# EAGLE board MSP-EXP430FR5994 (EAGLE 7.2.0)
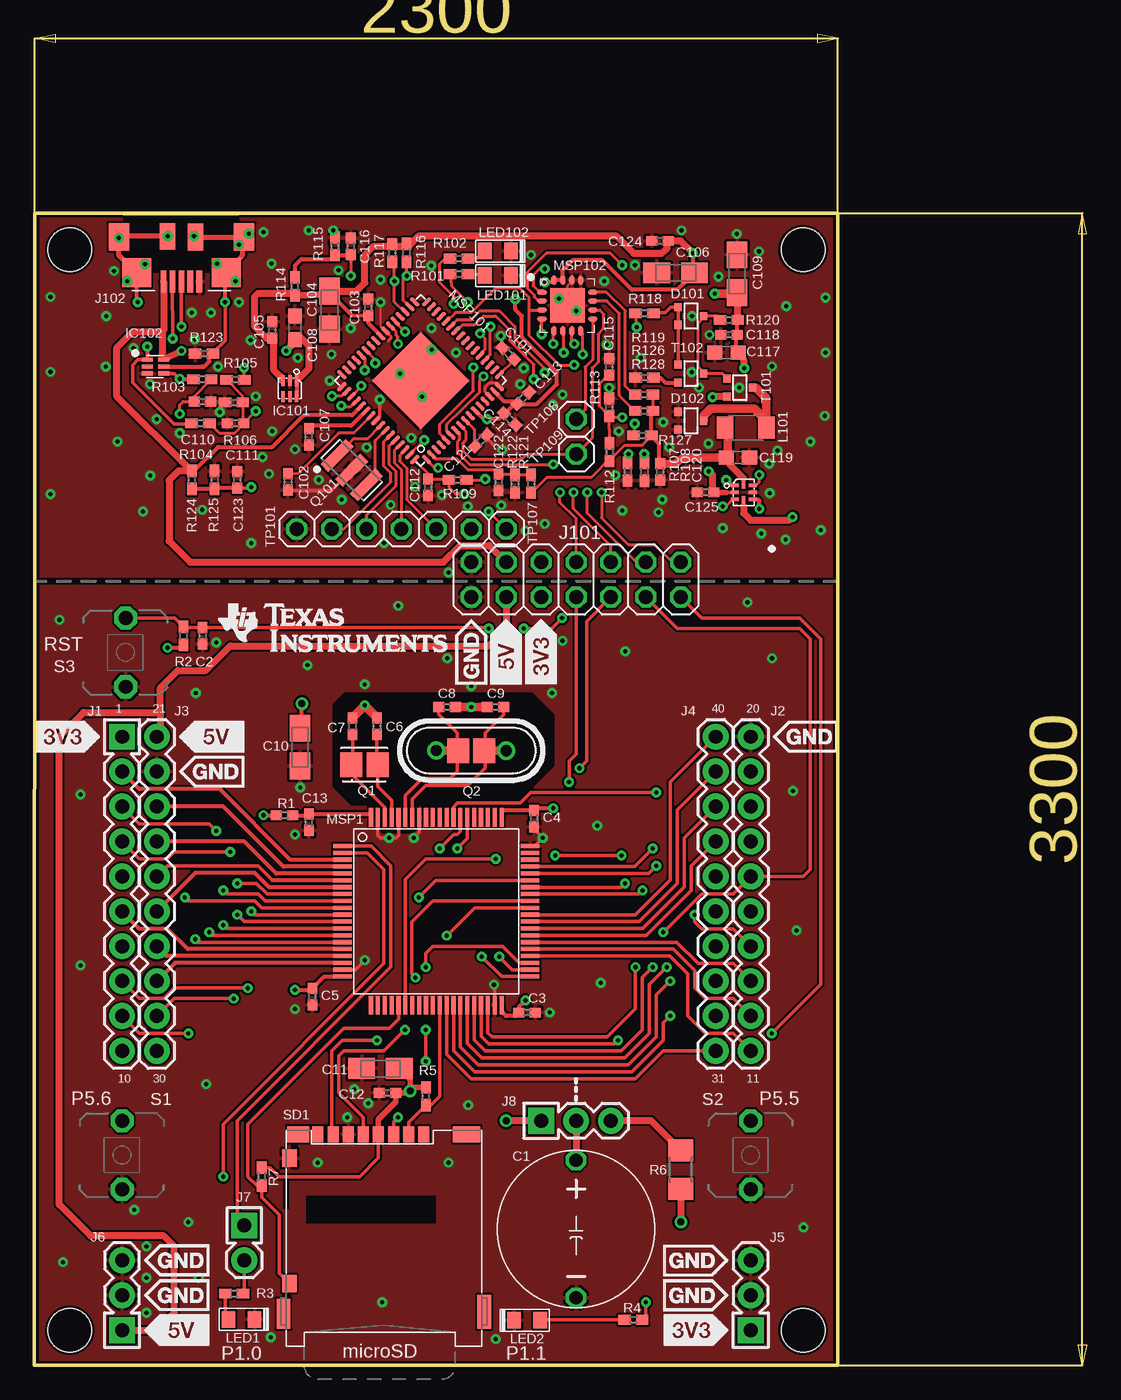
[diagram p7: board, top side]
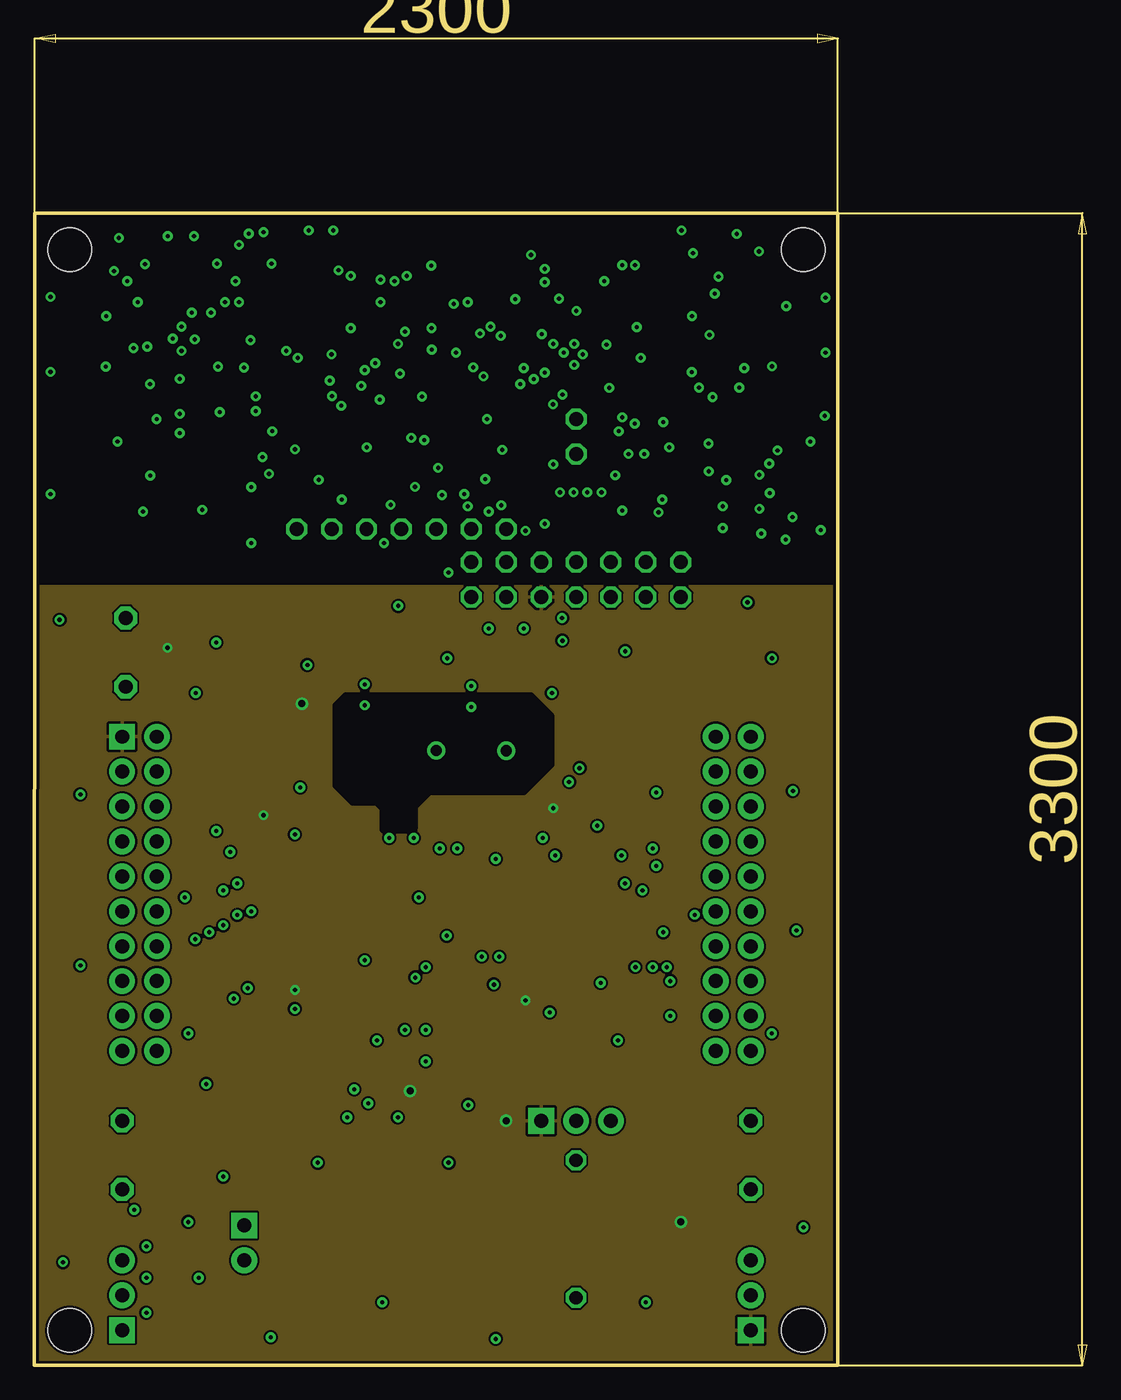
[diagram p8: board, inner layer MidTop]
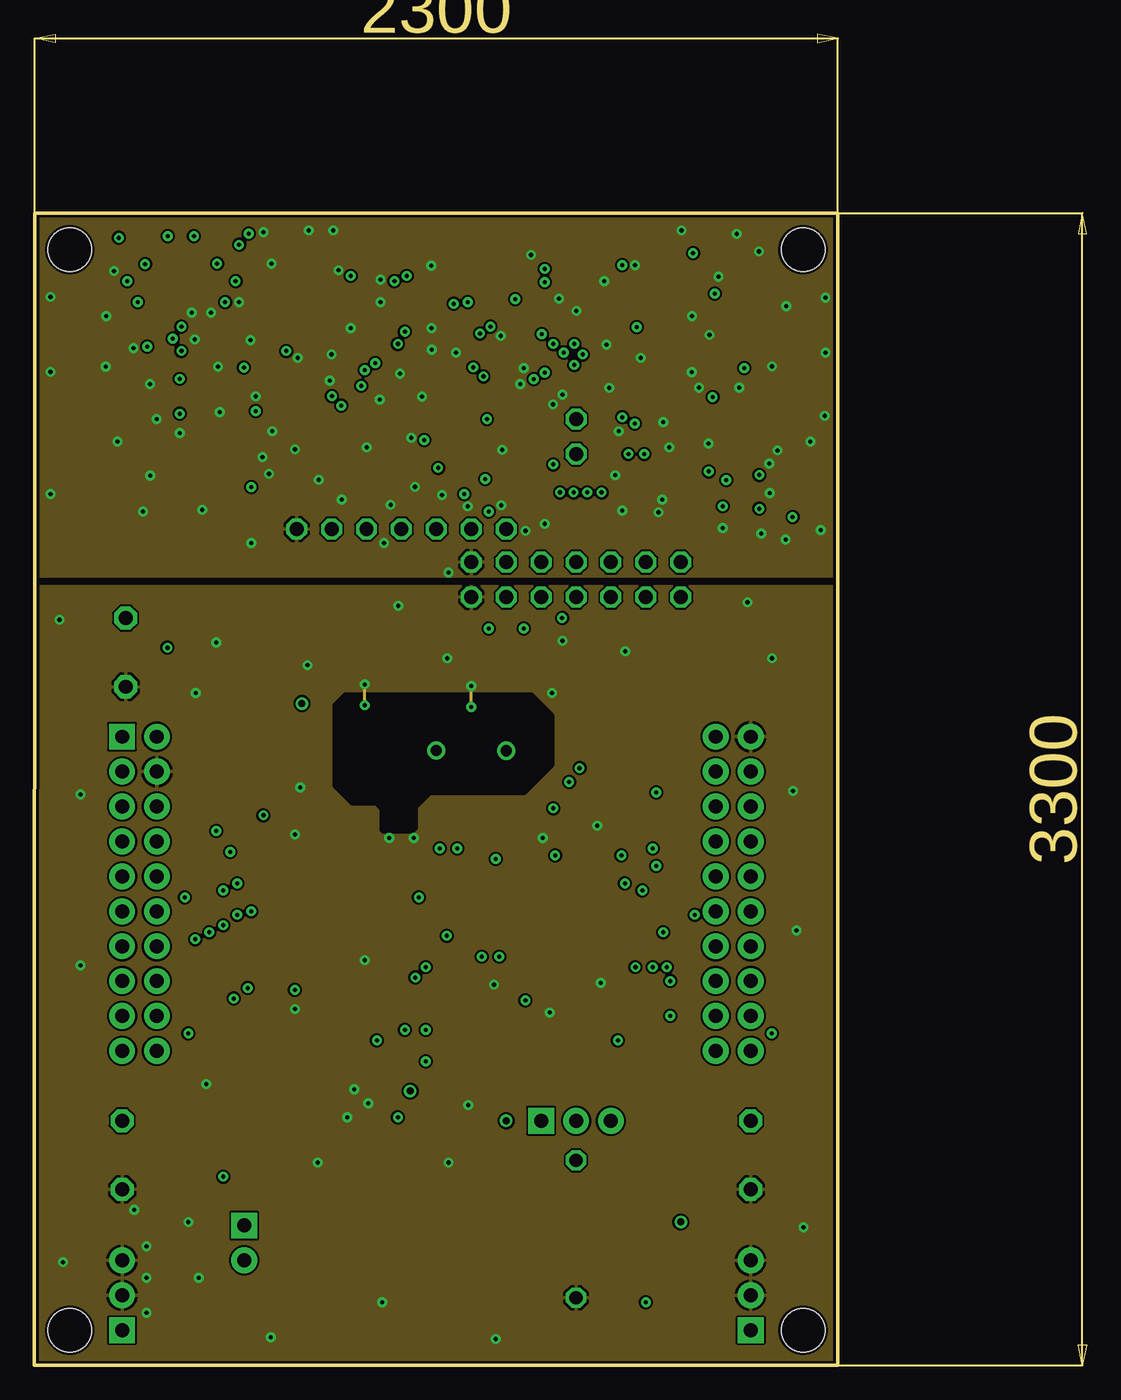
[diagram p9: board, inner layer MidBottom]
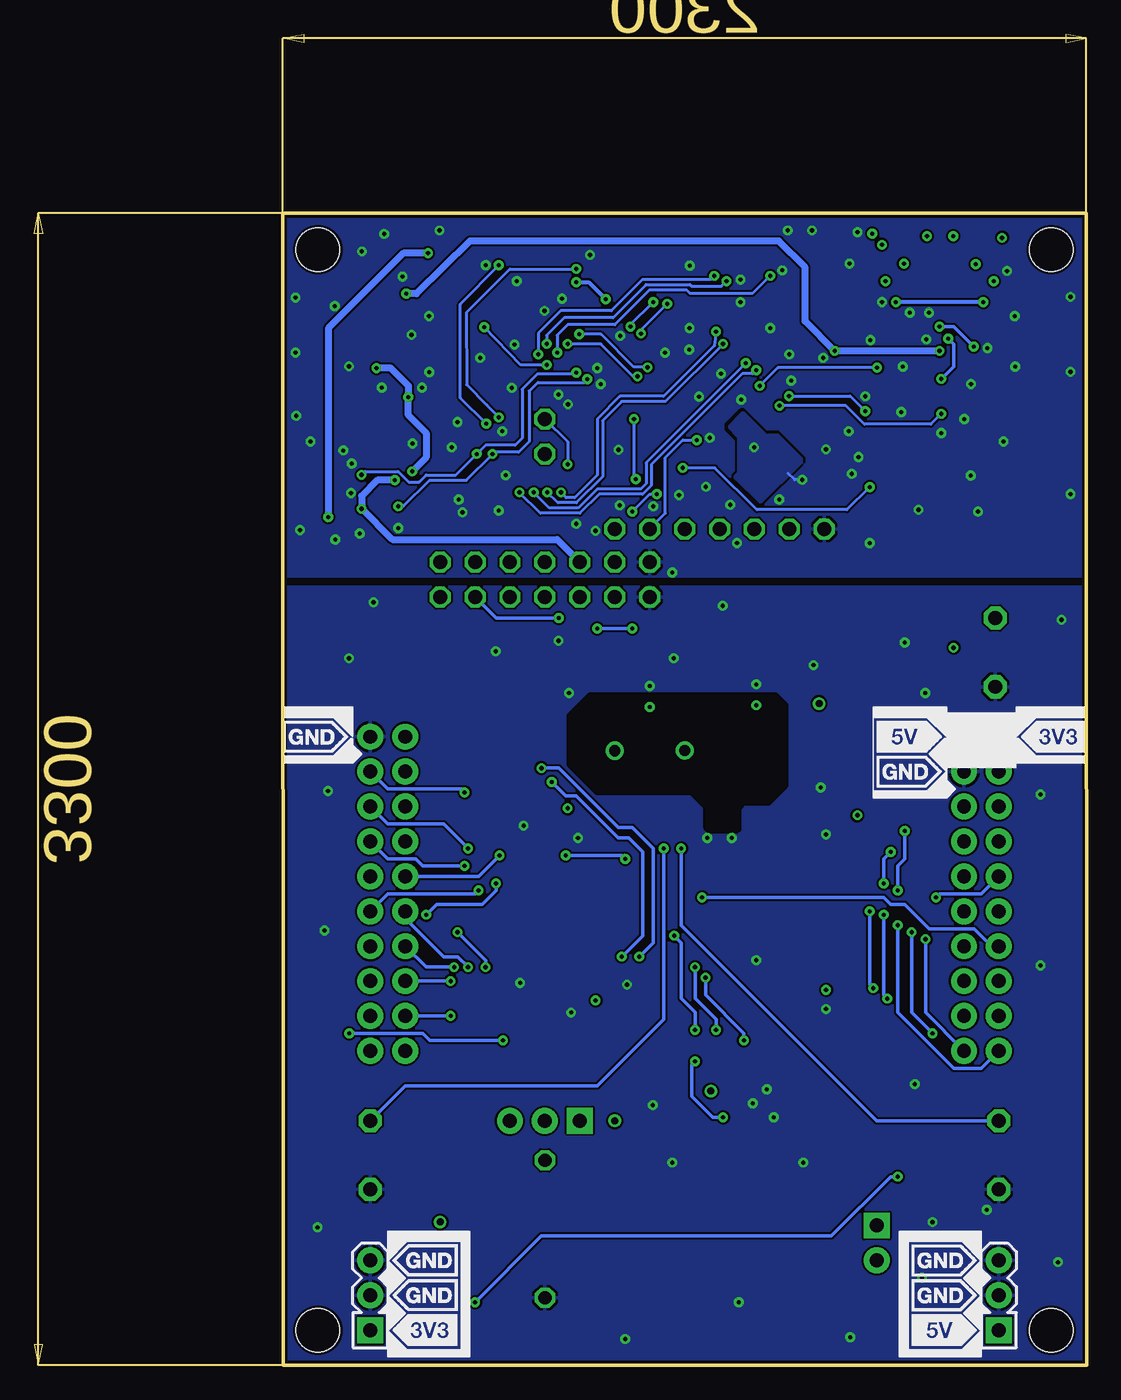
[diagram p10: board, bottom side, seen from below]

Size 76.53 x 96.82 mm. Coordinates in mm from the lower left corner, seen from the top.
Outline: 0,0 58.42,0 58.45,83.82 0.03,83.82 0,0
Copper layers (1+2*15+16): Top 0.0178mm / dielectric 12mil / MidTop 0.0356mm / dielectric 27mil / MidBottom 0.0356mm / dielectric 12mil / Bottom 0.0178mm
Design rules "MSP430 PCBExpress 4-layer-Stein": minimum track width 6mil, minimum drill 12mil, track to track 6mil, track to pad 6mil, pad to pad 6mil, via to via 8mil, smd to smd 6mil, copper to edge 8mil, drill to drill 8mil, minimum pad ring 10mil, minimum via ring 8mil, stop-mask expansion 8mil, vias tented up to drill 15mil, thermal gap 8mil
Net classes: 0 default: width 0.254 mm; 1 Ground: width 0.305 mm, drill 0.305 mm, clearance 0.152 mm to class 0, clearance 0.152 mm; 2 Power: width 0.406 mm, drill 0.305 mm, clearance 0.152 mm to class 0, clearance 0.152 mm to class 1, clearance 0.152 mm
tRestrict: area 20.5,62.5 to 26.3,69.6
bRestrict: area 20.5,62.5 to 26.3,69.6

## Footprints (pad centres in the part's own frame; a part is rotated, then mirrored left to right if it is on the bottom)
PANASONIC_SUPERCAP = drill 0.965 octagon: + 0,5; - 0,-5
0402 = smd 0.8 x 0.7: 1 -0.6,0; 2 0.6,0
A/3216-18R = smd 1.95 x 1.5: + 1.375,0; - -1.375,0
C0603 = smd 1.1 x 1: 1 -0.85,0; 2 0.85,0
SOT323 = smd 0.6 x 0.55: 1 -0.65,-0.825; 2 0.65,-0.825; 3 0,1.025
WSON_DSE = smd 0.25 x 0.8: 1 0,0; 2 0.5,0; 3 1,0; 5 0.5,1.15; 6 0,1.15; P4 1,1.15
SON(DRY)6 = smd 0.81 x 0.305: 1 -0.1,0; 2 -0.1,-0.5; 3 -0.1,-1; 4 1.1,-1; 5 1.1,-0.5; 6 1.1,0
UQFN_RSE = smd 0.25 x 0.58: 1 -0.5,-0.65; 2 0,-0.65; 3 0.5,-0.65; 5 0.5,0.65; 6 0,0.65; 7 -0.5,0.65 | smd 0.58 x 0.25: 4 0.55,0; 8 -0.55,0
J1 = drill 1.016 pad 1.88 square: 1 0,22.86 | drill 1.016 pad 1.88: 2 0,20.32; 3 0,17.78; 4 0,15.24; 5 0,12.7; 6 0,10.16; 7 0,7.62; 8 0,5.08; 9 0,2.54; 10 0,0
J2 = drill 1.016 pad 1.88: 11 0,0; 12 0,2.54; 13 0,5.08; 14 0,7.62; 15 0,10.16; 16 0,12.7; 17 0,15.24; 18 0,17.78; 19 0,20.32; 20 0,22.86
J3 = drill 1.016 pad 1.88: 21 0,22.86; 22 0,20.32; 23 0,17.78; 24 0,15.24; 25 0,12.7; 26 0,10.16; 27 0,7.62; 28 0,5.08; 29 0,2.54; 30 0,0
J4 = drill 1.016 pad 1.88: 31 0,0; 32 0,2.54; 33 0,5.08; 34 0,7.62; 35 0,10.16; 36 0,12.7; 37 0,15.24; 38 0,17.78; 39 0,20.32; 40 0,22.86
3PIN_PWR_3V3 = drill 1.016 pad 1.88 square: 1 0,0 | drill 1.016 pad 1.88: 2 0,2.54; 3 0,5.08
3PIN_PWR_5V = drill 1.016 pad 1.88 square: 1 0,0 | drill 1.016 pad 1.88: 2 0,2.54; 3 0,5.08
1X02 = drill 1.016 pad 1.88 square: 1 -1.27,0 | drill 1.016 pad 1.88: 2 1.27,0
1X03 = drill 1.016 pad 1.88 square: 1 0,0 | drill 1.016 pad 1.88: 2 2.54,0; 3 5.08,0
J101 = drill 1.016 octagon: 1 7.62,1.27; 2 7.62,-1.27; 3 5.08,1.27; 4 5.08,-1.27; 5 2.54,1.27; 6 2.54,-1.27; 7 0,1.27; 8 0,-1.27; 9 -2.54,1.27; 10 -2.54,-1.27; 11 -5.08,1.27; 12 -5.08,-1.27; 13 -7.62,1.27; 14 -7.62,-1.27
EZFET_UX62M-B-5P = smd 0.42 x 1.6: 1 1.3,1.3; 2 0.65,1.3; 3 0,1.3; 4 -0.65,1.3; 5 -1.3,1.3 | smd 2.1 x 2.1: S1 -3.25,0.65; S2 3.25,0.65 | smd 1.5 x 2: S3 -4.55,-1.95; S4 4.55,-1.95 | smd 1.144 x 1.949: S5 -1.016,-1.93; S6 1.016,-1.981
L3216C = smd 1.2 x 1.6: 1 -1.5,0; 2 1.5,0
LED0805 = smd 1 x 1.2: A 1.052,0.102; C -0.848,0.102
PN80 = smd 1.35 x 0.3: 1 -6.825,4.75; 2 -6.825,4.25; 3 -6.825,3.75; 4 -6.825,3.25; 5 -6.825,2.75; 6 -6.825,2.25; 7 -6.825,1.75; 8 -6.825,1.25; 9 -6.825,0.75; 10 -6.825,0.25; 11 -6.825,-0.25; 12 -6.825,-0.75; 13 -6.825,-1.25; 14 -6.825,-1.75; 15 -6.825,-2.25; 16 -6.825,-2.75; 17 -6.825,-3.25; 18 -6.825,-3.75; 19 -6.825,-4.25; 20 -6.825,-4.75; 41 6.825,-4.75; 42 6.825,-4.25; 43 6.825,-3.75; 44 6.825,-3.25; 45 6.825,-2.75; 46 6.825,-2.25; 47 6.825,-1.75; 48 6.825,-1.25; 49 6.825,-0.75; 50 6.825,-0.25; 51 6.825,0.25; 52 6.825,0.75; 53 6.825,1.25; 54 6.825,1.75; 55 6.825,2.25; 56 6.825,2.75; 57 6.825,3.25; 58 6.825,3.75; 59 6.825,4.25; 60 6.825,4.75 | smd 0.3 x 1.35: 21 -4.75,-6.825; 22 -4.25,-6.825; 23 -3.75,-6.825; 24 -3.25,-6.825; 25 -2.75,-6.825; 26 -2.25,-6.825; 27 -1.75,-6.825; 28 -1.25,-6.825; 29 -0.75,-6.825; 30 -0.25,-6.825; 31 0.25,-6.825; 32 0.75,-6.825; 33 1.25,-6.825; 34 1.75,-6.825; 35 2.25,-6.825; 36 2.75,-6.825; 37 3.25,-6.825; 38 3.75,-6.825; 39 4.25,-6.825; 40 4.75,-6.825; 61 4.75,6.825; 62 4.25,6.825; 63 3.75,6.825; 64 3.25,6.825; 65 2.75,6.825; 66 2.25,6.825; 67 1.75,6.825; 68 1.25,6.825; 69 0.75,6.825; 70 0.25,6.825; 71 -0.25,6.825; 72 -0.75,6.825; 73 -1.25,6.825; 74 -1.75,6.825; 75 -2.25,6.825; 76 -2.75,6.825; 77 -3.25,6.825; 78 -3.75,6.825; 79 -4.25,6.825; 80 -4.75,6.825
RGC64 = smd 0.825 x 0.28: 1 -4.36,3.75; 2 -4.36,3.25; 3 -4.36,2.75; 4 -4.36,2.25; 5 -4.36,1.75; 6 -4.36,1.25; 7 -4.36,0.75; 8 -4.36,0.25; 9 -4.36,-0.25; 10 -4.36,-0.75; 11 -4.36,-1.25; 12 -4.36,-1.75; 13 -4.36,-2.25; 14 -4.36,-2.75; 15 -4.36,-3.25; 16 -4.36,-3.75; 33 4.36,-3.75; 34 4.36,-3.25; 35 4.36,-2.75; 36 4.36,-2.25; 37 4.36,-1.75; 38 4.36,-1.25; 39 4.36,-0.75; 40 4.36,-0.25; 41 4.36,0.25; 42 4.36,0.75; 43 4.36,1.25; 44 4.36,1.75; 45 4.36,2.25; 46 4.36,2.75; 47 4.36,3.25; 48 4.36,3.75 | smd 0.28 x 0.825: 17 -3.75,-4.36; 18 -3.25,-4.36; 19 -2.75,-4.36; 20 -2.25,-4.36; 21 -1.75,-4.36; 22 -1.25,-4.36; 23 -0.75,-4.36; 24 -0.25,-4.36; 25 0.25,-4.36; 26 0.75,-4.36; 27 1.25,-4.36; 28 1.75,-4.36; 29 2.25,-4.36; 30 2.75,-4.36; 31 3.25,-4.36; 32 3.75,-4.36; 49 3.75,4.36; 50 3.25,4.36; 51 2.75,4.36; 52 2.25,4.36; 53 1.75,4.36; 54 1.25,4.36; 55 0.75,4.36; 56 0.25,4.36; 57 -0.25,4.36; 58 -0.75,4.36; 59 -1.25,4.36; 60 -1.75,4.36; 61 -2.25,4.36; 62 -2.75,4.36; 63 -3.25,4.36; 64 -3.75,4.36 | smd 5 x 5: TP 0,0
RSA16 = smd 0.7 x 0.35: 1 -1.85,0.975; 2 -1.85,0.325; 3 -1.85,-0.325; 4 -1.85,-0.975; 9 1.85,-0.975; 10 1.85,-0.325; 11 1.85,0.325; 12 1.85,0.975 | smd 0.35 x 0.7: 5 -0.975,-1.85; 6 -0.325,-1.85; 7 0.325,-1.85; 8 0.975,-1.85; 13 0.975,1.85; 14 0.325,1.85; 15 -0.325,1.85; 16 -0.975,1.85 | smd 2.5 x 2.5: TP 0,0
LF_CRYSTAL = smd 1.778 x 1.6: 1 0,0.94; 2 0,-0.965
HF_XTAL = drill 0.813: 1 0.009,2.543; 2 -0.001,-2.533 | smd 1.8 x 1.6: P$1 0,-0.95; P$2 0,0.95
CSTCR4M = smd 0.8 x 2.6: 1 -1.5,0; 2 0,0; 3 1.5,0
0402' = smd 0.9 x 0.7: 1 -0.65,0; 2 0.65,0
R3216 = smd 1.6 x 1.8: 1 -1.4,0; 2 1.4,0
PBTH = drill 1.016 pad 1.676 octagon: 1 -0.001,0.001; 2 5.001,0.001
SD-502702-003 = smd 0.8 x 1.16: 1 -2.9,-17.82; 2 -1.8,-17.82; 3 -0.7,-17.82; 4 0.4,-17.82; 5 1.5,-17.82; 6 2.6,-17.82; 7 3.7,-17.82; 8 4.8,-17.82 | smd 1.05 x 1.25: A 6.885,-16.075; B 6.885,-6.95 | smd 1 x 2.5: P$9 -7.3,-4.9 | smd 1 x 2.2: P$10 7.3,-4.75 | smd 2 x 1.16: P$11 -6.01,-17.82 | smd 1.6 x 1.16: P$12 6.24,-17.82
1X01 = drill 1.016 octagon: 1 0,0
MOUNTHOLE_125MIL = hole 3.175: 0,0

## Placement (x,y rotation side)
C1  0.1F  [PANASONIC_SUPERCAP]  39.4,9.91 0 top
C2  1n  [0402]  12.24,53.07 270 top
C3  100n  [0402]  35.84,25.65 0 top
C4  100n  [0402]  36.35,39.75 270 top
C5  100n  [0402]  20.22,26.8 270 top
C6  22p  [0402]  24.92,46.48 90 top
C7  22p  [0402]  23.14,46.48 90 top
C8  DNP  [0402]  30,47.88 0 top
C9  DNP  [0402]  33.55,47.88 180 top
C10  10u  [A/3216-18R]  19.33,44.96 90 top
C11  1u  [A/3216-18R]  25.17,21.59 0 top
C12  100n  [0402]  25.68,19.81 180 top
C13  100n  [0402]  19.96,39.5 270 top
C101  470n  [0402]  34.46,73.6 135 top
C102  220n  [0402]  18.44,64.26 270 top
C103  100n  [0402]  24.28,76.96 90 top
C104  10u  [A/3216-18R]  21.46,76.76 90 top
C105  100n  [0402]  17.3,75.31 90 top
C106  4.7u  [A/3216-18R]  46.63,79.47 0 top
C107  220n  [0402]  19.96,67.54 270 top
C108  1u  [C0603]  18.95,75.46 90 top
C109  4.7u  [A/3216-18R]  51.11,79.4 270 top
C110  10p  [0402]  12.22,70.1 0 top
C111  10p  [0402]  14.63,68.52 180 top
C112  1n  [0402]  28.64,63.85 270 top
C113  100n  [0402]  35.55,70.36 45 top
C114  100n  [0402]  34.57,68.83 315 top
C115  33p  [0402]  41.81,72.64 270 top
C116  33p  [0402]  23.01,81.41 270 top
C117  4.7u  [C0603]  50.33,73.67 180 top
C118  100n  [0402]  50.51,74.97 180 top
C119  4.7u  [C0603]  51.16,66.03 0 top
C120  100n  [0402]  45.52,64.99 270 top
C121  100n  [0402]  32.48,67.26 45 top
C122  33p  [0402]  33.77,64.21 90 top
C123  33p  [0402]  14.76,64.41 270 top
C124  100n  [0402]  45.49,81.79 180 top
C125  100n  [0402]  48.79,63.5 180 top
D101  BAS40-05  [SOT323]  47.65,76.33 270 top
D102  BAS40-05  [SOT323]  47.65,68.71 270 top
DRAW1  [LOGO-ROCKET-10X7MM-BRD]  2.84,63.13 56 top
DRAW3  [LOGO-ROCKET-10X7MM-BRD]  10.52,15.59 7 top
IC101  [WSON_DSE]  19.08,71.63 180 top
IC102  TPD4E004DRYR  [SON(DRY)6]  8.31,73.15 0 top
IC103  TS5A21366RSER  [UQFN_RSE]  51.59,63.5 270 top
J1  BP_HEADERS_J1  [J1]  6.38,22.86 0 top
J2  BP_HEADERS_J2  [J2]  52.1,22.86 0 top
J3  BP_HEADERS_J3  [J3]  8.92,22.86 0 top
J4  BP_HEADERS_J4  [J4]  49.56,22.86 0 top
J5  HEADER 1X03  [3PIN_PWR_3V3]  52.1,2.54 0 bottom
J6  BP_HEADERS_PWR_5V  [3PIN_PWR_5V]  6.38,2.54 0 bottom
J7  JUMPER1X02  [1X02]  15.27,8.89 270 top
J8  JUMPER1X03  [1X03]  36.86,17.78 0 top
J101  J101_2X7_HEADER  [J101]  39.4,57.15 0 top
J102  Micro-USB  [EZFET_UX62M-B-5P]  10.69,80.14 180 top
L101  2u2  [L3216C]  51.73,68.19 180 top
LED1  Red  [LED0805]  15.16,3.43 180 top
LED2  Green  [LED0805]  35.74,3.17 0 top
LED101  Red  [LED0805]  33.81,79.38 180 top
LED102  Green  [LED0805]  33.81,81.15 180 top
MSP1  MSP430FR5994  [PN80]  29.24,33.02 0 top
MSP101  MSP430F5528IRGC  [RGC64]  28.09,71.63 135 top
MSP102  MSP430G2452IRSA16R  [RSA16]  38.76,77.09 0 top
Q1  LF_CRYSTAL  [LF_CRYSTAL]  24.03,43.69 270 top
Q2  [HF_XTAL]  31.78,44.7 90 top
Q101  PIEZO_CSTCR4M00G15L99  [CSTCR4M]  23.08,65.11 315 top
R1  0R  [0402]  18.19,40.01 0 top
R2  47k  [0402']  10.84,53.07 270 top
R3  470  [0402']  14.53,5.21 180 top
R4  390  [0402']  43.56,3.3 180 top
R5  47k  [0402']  28.47,19.56 90 top
R6  22  [R3216]  47.02,14.22 90 top
R7  DNP- 100k  [0402']  16.54,13.72 270 top
R101  470  [0402']  30.89,79.38 180 top
R102  390  [0402']  30.89,80.5 180 top
R103  27  [0402']  12.22,71.72 0 top
R104  27  [0402']  12.09,68.52 0 top
R105  1k4  [0402']  14.63,71.69 0 top
R106  1M  [0402']  14.5,70.04 180 top
R107  47k  [0402']  43.15,65 270 top
R108  47k  [0402']  44.37,65 270 top
R109  47k  [0402']  30.79,64.4 0 top
R112  220k  [0402']  41.84,66.42 90 top
R113  220k  [0402']  41.81,69.7 90 top
R114  220k  [0402']  18.95,78.49 90 top
R115  220k  [0402']  21.87,81.41 90 top
R116  4k7  [0402']  27.06,80.91 270 top
R117  4k7  [0402']  26.03,80.91 270 top
R118  820  [0402']  44.37,76.52 180 top
R119  0  [0402']  44.37,71.84 180 top
R120  470  [0402']  50.51,76.03 180 top
R121  220k  [0402']  36.13,64.14 90 top
R122  220k  [0402']  34.95,64.14 270 top
R123  33k  [0402']  12.34,73.6 180 top
R124  240k  [0402']  11.46,64.41 270 top
R125  150k  [0402']  13.11,64.41 90 top
R126  2k2  [0402']  44.35,70.61 180 top
R127  3k3  [0402']  44.22,67.64 180 top
R128  6k8  [0402']  44.35,69.42 180 top
S1  [PBTH]  6.38,17.78 270 top
S2  [PBTH]  52.1,17.78 270 top
S3  [PBTH]  6.63,54.36 270 top
SD1  SD-502702-003-1  [SD-502702-003]  25.43,-1.02 180 top
T101  DMG1013UW  [SOT323]  51.21,71.12 270 top
T102  BC850CW-115  [SOT323]  47.65,72.14 270 top
TP101  TEST_PIN2  [1X01]  19.08,60.83 0 top
TP102  TEST_PIN2  [1X01]  21.62,60.83 0 top
TP103  TEST_PIN2  [1X01]  24.16,60.83 0 top
TP104  TEST_PIN2  [1X01]  26.7,60.83 0 top
TP105  TEST_PIN2  [1X01]  29.24,60.83 0 top
TP106  TEST_PIN2  [1X01]  31.78,60.83 0 top
TP107  TEST_PIN2  [1X01]  34.32,60.83 0 top
TP108  TEST_PIN2  [1X01]  39.4,68.83 0 top
TP109  TEST_PIN2  [1X01]  39.4,66.29 0 top
U$1  FR5994_REARSILK_REV1_0  [FR5994_REARSILK_REV1_0]  0.03,0 0 top
U$2  MOUNTHOLE_125MIL  [MOUNTHOLE_125MIL]  2.57,2.54 0 top
U$3  MOUNTHOLE_125MIL  [MOUNTHOLE_125MIL]  2.57,81.15 0 top
U$4  [LOGO16_TPLACE]  13.28,51.73 0 top
U$5  MOUNTHOLE_125MIL  [MOUNTHOLE_125MIL]  55.91,2.54 0 top
U$6  MOUNTHOLE_125MIL  [MOUNTHOLE_125MIL]  55.91,81.15 0 top
U$7  MIKE_TM  [MIKE_TM]  25.17,8.13 0 top
U$8  BP_3PIN_SILK  [3PIN_PWR_SILK]  7.65,0.61 0 top
U$10  BP_3PIN_SILK_RT  [3PIN_PWR_SILK_RT]  50.83,0.61 0 top

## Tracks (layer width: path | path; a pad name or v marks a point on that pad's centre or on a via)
!RST!/SBWTDIO  (via drill 0.3)
  Top 0.203: R2.1 10.9,53.67
  Top 0.254: R2.1 10.2,54.36 S3.1 | 10.9,53.67 C2.1 32.97,53.67 v33.05,53.59 | v35.59,53.59 37.62,53.59 v38.38,54.36 | J101.4 46.76,53.59 55.65,53.59 56.41,52.83 56.41,36.07 55.91,35.56 J2.16 50.83,34.29 48.54,34.29 v45.75,31.5 | MSP1.38 32.99,24.19 33.3,23.88 41.68,23.88 43.71,25.91 v43.71,28.96
  Bottom 0.254: v33.05,53.59 v35.59,53.59 | v38.38,54.36 42.95,54.36 J101.4 | v43.71,28.96 43.71,29.46 v45.75,31.5
+3V3  (via drill 0.3, 0.51)
  Top 0.203: 10.84,52.35 R2.2
  Top 0.254: SD1.4 25.03,15.09 23.65,13.72 17.81,13.72 17.16,14.37 R7.1
  Top 0.305: v9.68,52.2 10.62,52.2 R2.2 | 33.99,25.91 MSP1.40 33.99,25.73 34.32,25.4 34.99,25.4 C3.1 35.24,26.07 v35.71,26.54 | v18.95,27.3 20.22,27.3 C5.1 21.09,28.27 MSP1.20 | MSP1.61 33.99,40.35 C4.1 36.35,40.51 v37.74,40.51 | v16.66,40.01 R1.1 | C10.+ 19.46,46.33 v19.46,48.13
  Top 0.406: J1.1 6.38,45.64 | R5.2 27.6,20.21 v27.33,19.94 | SD1.4 25.03,17.89 26.28,19.14 C12.1 27.2,19.81 v27.33,19.94 | 27.33,20.28 v27.33,19.94 | C11.+ 27.33,20.81 v27.33,19.94
  Top 0.508: R6.1 v47.02,10.41 | J8.1 v34.32,17.78
  pour MidTop: 0.03,56.64 0.03,0 58.45,0 58.45,56.64
+5V
  Top 0.508: J101.12 34.32,53.59 33.05,52.32 14.25,52.32 12.47,50.55 10.44,50.55 9.17,49.28 9.17,47.5 | J6.1 8.92,2.54 10.19,3.81 10.19,8.64 9.42,9.4 4.09,9.4 1.8,11.68 1.8,45.72 3.58,47.5 9.17,47.5 | 9.17,47.5 9.17,45.97 J3.21
EZFET_AVBUS  (via drill 0.3)
  Top 0.203: v29.36,65.28 29.11,65.28 28.52,65.86 MSP101.1
  Top 0.254: C123.2 15.71,63.81 v15.77,63.88
  Top 0.305: 12.96,63.86 12.98,63.88 13.12,63.88 | 13.11,63.86 R125.1 | 13.23,63.88 13.12,63.88 | 13.12,63.88 R125.1 | R124.2 R125.1 | R125.1 | C123.2 13.16,63.81 R125.1
  Bottom 0.203: v29.36,65.28 27.03,65.28 23.98,62.23 17.42,62.23 v15.77,63.88
EZFET_AVCC  (via drill 0.3)
  Top 0.152: 38.51,75.17 38.51,75.18 MSP102.6
  Top 0.203: 23.01,80.38 v23.01,79.25 | v38.51,73.66 38.51,75.17
  Top 0.305: 23.01,80.38 C116.2 | 22.97,80.48 23.01,80.52 23.01,80.48 | 23.01,80.39 23.01,80.48 | 23.01,80.48 C116.2 | R114.2 18.95,79.04 18.95,80.01 19.41,80.48 21.59,80.48 R115.1 22.96,80.76 C116.2
  Bottom 0.203: v23.01,79.25 24.28,77.98 28.85,77.98 29.11,78.23 31.78,78.23 34.32,75.69 37.74,75.69 38.51,74.93 v38.51,73.66
EZFET_AVCCOUT  (via drill 0.3)
  Top 0.152: 36.73,78.11 36.86,78.11 MSP102.1
  Top 0.203: R113.1 41.81,68.08 41.81,68.07 41.81,67.06 41.83,67.06 R112.2 | R113.1 42.03,68.96 v42.75,68.96 | 36.73,78.11 36.27,78.54 36.27,79.3 36.73,79.76 v37.11,79.76 | 41.78,72.06 41.78,72.03 41.83,71.98 41.83,71.99 41.86,72.01 | 41.86,71.92 41.86,72.01 | 41.86,72.01 41.86,72.04 41.83,72.06 | C115.2 41.79,72.09 41.07,71.37 41.07,69.8 41.68,69.19 41.77,68.94 R113.1
  Top 0.508: C115.2 41.81,72.08 41.78,72.06
  Bottom 0.203: v37.11,79.76 41.94,79.76 45.11,76.58 45.09,71.32 43.61,69.85 v42.75,68.96
EZFET_AVCCOUT2ADC
  Top 0.203: MSP101.2 29.21,65.91 30.76,65.91 31.52,65.15 33.43,65.15 C122.2 34.92,64.81 R122.1 R121.2 | R121.2
EZFET_DCDCCAL0
  Top 0.203: R126.2 43.7,70.48 43.33,70.87 42.98,71.22 42.98,76.71 41.6,78.06 MSP102.12
EZFET_DCDCCAL1  (via drill 0.3)
  Top 0.203: MSP102.2 36.85,77.47 36.6,77.47 36.35,77.72 36.35,77.85 35.84,78.36 35.84,79.5 37.24,80.9 41.88,80.9 v42.75,80.03 | R127.2 43.67,67.61 43.66,67.97 43.66,68.43 43.69,68.45 43.66,68.45 v43.66,68.5
  Bottom 0.203: v42.75,80.03 45.54,77.19 45.54,70.36 v43.66,68.5
EZFET_DCDCCAL2
  Top 0.203: MSP102.11 40.63,77.42 41.63,77.42 42.55,76.5 42.55,70.55 43.67,69.42 R128.2
EZFET_DCDCIO0  (via drill 0.3)
  Top 0.203: v36.91,75.01 36.91,75.24 MSP102.4 | v31.93,72.59 31.93,70.89 29.49,68.45 29.49,67.76 MSP101.5
  Bottom 0.203: v36.91,75.01 35.31,75.01 32.92,72.62 32.16,72.62 v31.93,72.59
EZFET_DCDCIO1  (via drill 0.3)
  Top 0.203: 30.12,67.83 MSP101.6 30,67.96 30,68.45 32.35,70.75 32.36,70.77 32.36,71.63 v32.66,71.93 | v37.74,74.3 37.74,75.2 MSP102.5
  Bottom 0.203: v37.74,74.3 35.33,74.3 32.97,71.93 v32.66,71.93
EZFET_DCDCPULSE  (via drill 0.3)
  Top 0.203: R118.2 43.82,75.81 v43.82,75.51 | v39.27,72.77 38.18,72.77 35.97,74.93 35.97,76.84 | 35.97,76.84 35.97,77.7 35.31,78.36 33.55,78.36 31.78,76.58 30.63,76.58 30,75.95 MSP101.28 | 35.97,76.84 36.04,76.76 MSP102.3
  Bottom 0.203: v39.27,72.77 41.15,72.77 v43.82,75.51
EZFET_DCDCRST  (via drill 0.3)
  Top 0.203: MSP101.7 30.66,67.99 30.91,67.74 30.91,67.33 30.76,67.18 30.76,66.42 31.65,65.53 v37.74,65.53 | 40.78,76.07 MSP102.9 40.61,73.17 40.06,72.62 40.06,69.52 TP108.1 | TP108.1 39.42,68.86 39.37,68.91 TP108.1
  Top 0.305: TP108.1
  Bottom 0.203: TP108.1 | TP108.1 37.74,67.18 v37.74,65.53
EZFET_DCDCTEST
  Top 0.203: MSP101.8 31,68.34 31.37,67.97 31.37,67.28 31.14,67.06 31.14,66.55 31.78,65.91 35.46,65.91 35.84,66.29 TP109.1 39.8,66.7 40.56,67.46 40.56,72.54 41,72.97 41,75.01 41.43,75.44 41.43,76.45 41.12,76.76 40.74,76.76 40.67,76.83 40.67,76.71 MSP102.10
EZFET_DM  (via drill 0.3)
  Top 0.203: J102.2 10.04,78.75
  Top 0.254: IC102.4 10.17,72.15 v10.57,71.75 | 10.04,78.75 v10.06,74.68
  Top 0.305: v10.57,71.75 11.58,71.75 11.61,71.72 R103.1
  Bottom 0.254: v10.57,71.75 9.68,72.64 9.68,74.3 v10.06,74.68
EZFET_DP  (via drill 0.3)
  Top 0.254: v8.2,74.09 v8.21,74.1 IC102.1 7.52,73.15 7.14,72.77 7.14,71.5 10.19,68.45 11.5,68.45 R104.1 | J102.3 v10.69,75.56
  Bottom 0.254: v10.69,75.56 9.68,75.56 v8.2,74.09
EZFET_HOSTSCL  (via drill 0.3)
  Top 0.152: MSP101.35 26.95,76.71 26.95,76.7
  Top 0.203: 26.95,76.7 26.83,76.7 26.19,77.34 v26.19,78.87 26.19,80.34 | v39.27,74.3 39.09,74.45 MSP102.7
  Top 0.305: 26.19,80.34 R117.2
  Bottom 0.203: v26.19,78.87 26.57,78.49 28.73,78.49 28.85,78.61 32.03,78.61 34.44,76.2 38,76.2 39.27,74.93 v39.27,74.3
EZFET_HOSTSDA  (via drill 0.3)
  Top 0.203: MSP101.34 27.28,77.01 26.82,77.47 26.82,78.99 v27.08,79.25 27.08,80.25 R116.2 | MSP102.8 39.88,75.07 v39.88,73.53
  Bottom 0.203: v27.08,79.25 27.33,78.99 32.28,78.99 34.57,76.71 38.25,76.71 39.88,75.08 v39.88,73.53
EZFET_LED0  (via drill 0.3)
  Top 0.203: MSP101.20 33.17,73.53 v33.17,75.56 | v31.52,77.34 30.34,78.53 R101.2
  Bottom 0.203: v33.17,75.56 33.17,75.69 v31.52,77.34
EZFET_LED1  (via drill 0.3)
  Top 0.203: 30.24,80.38 R102.2 29.85,80.5 29.49,80.14 29.49,78.74 30.51,77.72 v30.51,77.22 | MSP101.21 32.41,73.54 32.79,73.91 32.79,74.68 v32.41,75.06
  Bottom 0.203: v32.41,75.06 32.41,75.31 v30.51,77.22
EZFET_PU.0/DP  (via drill 0.3)
  Top 0.152: 22.76,70.87 MSP101.50
  Top 0.203: v16.1,69.42 15.33,68.64 C111.1 | R104.2 13.39,67.87 13.46,67.79 14.56,67.79 C111.1 | 15.15,68.44 C111.1 | 22.76,70.87 22.5,70.61 22.45,70.61 22.35,70.51 v21.64,70.51 | 15.18,68.62 C111.1 | R105.1 15.15,70.52 R106.1 15.15,68.59 C111.1
  Bottom 0.203: v16.1,69.42 17.2,70.51 v21.64,70.51
EZFET_PU.1/DM  (via drill 0.3)
  Top 0.203: 12.74,71.66 R103.2 11.62,70.47 C110.1 10.82,70.1 10.57,69.85 v10.57,69.22 | MSP101.52 23.01,69.72 22.5,69.72 v22.33,69.8
  Bottom 0.203: v22.33,69.8 17.5,69.8 16.15,68.45 11.33,68.45 v10.57,69.22
EZFET_PUR  (via drill 0.3)
  Top 0.203: MSP101.51 23.52,70.94 v23.77,71.25 | v15.24,72.57 15.25,71.79 R105.2
  Bottom 0.203: v15.24,72.57 22.45,72.57 v23.77,71.25
EZFET_RST  (via drill 0.3)
  Top 0.203: MSP101.64 27.79,65.71 28.64,64.86 C112.1 | 28.6,64.47 C112.1 | C112.1 30.09,64.45 R109.1 30.14,63.87 30.63,63.37 v31.27,63.37 | TP107.1 | TP107.1 v33.05,62.1
  Bottom 0.203: v33.05,62.1 31.78,63.37 v31.27,63.37
EZFET_SBWTCK  (via drill 0.3)
  Top 0.203: MSP101.44 23.75,73.48 24.03,73.2 v24.03,72.39 | v41.25,63.5 41.25,61.65 43.18,59.72 45.09,59.72 46.38,58.42 J101.1
  Bottom 0.203: v24.03,72.39 24.28,72.14 25.04,72.14 31.65,65.53 31.65,64.01 32.28,63.37 35.46,63.37 36.86,61.98 39.73,61.98 v41.25,63.5
EZFET_SBWTDIO  (via drill 0.3)
  Top 0.203: MSP101.43 24.13,73.82 24.79,73.15 v24.79,72.9 | J101.3 43.79,58.42 42.55,59.66 42.52,59.66 40.21,61.98 v40.21,63.5
  Bottom 0.203: v24.79,72.9 32.03,65.66 32.03,64.14 32.41,63.75 35.59,63.75 36.98,62.36 39.07,62.36 v40.21,63.5
EZFET_SHIELD  (via drill 0.3)
  Top 0.152: 14,79.12 13.87,78.99 13.87,78.87
  Top 0.203: 7.44,77.22 7.52,77.22 v7.52,77.34 | 7.44,78.87 7.39,78.87 | 7.39,78.87 7.39,79.38 | v6.76,78.87 7.39,78.87 | v14.63,78.87 13.87,78.87
  Top 0.254: R123.1 12.92,73.6 13.87,74.55 v13.87,77.34
  Top 0.305: IC102.5 12.21,72.65 12.34,72.64 12.73,73.03 12.73,73.43 R123.1 12.73,73.33 | 7.44,77.22 7.44,78.87 | v13.87,77.34 13.87,78.87
  Top 0.381: J102.S2 7.41,79.49 6.12,80.77 6.12,82.04 6.14,82.06 J102.S4 | J102.S4 v6.14,82.02 v6.15,82.02 | 14,79.12 14,79.54 | J102.S2 7.44,79.43 7.39,79.38 | v8.05,80.11 8.05,80.09 J102.S2 | v13.28,80.14 v13.29,80.14 J102.S1 14,79.54 | 14,79.54 14,79.63 15.14,80.77 15.14,81.25 v14.88,81.51 14.88,81.73 J102.S3 | v15.6,82.32 15.6,82.06 J102.S3 | J102.S3 15.22,82.07 J102.S5 11.68,82.07 v11.61,82.14 | 9.68,82.14 6.2,82.14 J102.S4
  Top 0.406: J102.S6 9.68,82.14 v9.7,82.14
  Bottom 0.305: v7.52,77.34 v13.87,77.34
EZFET_TCK  (via drill 0.3)
  Top 0.203: v28.35,67.31 27.31,66.27 MSP101.63
  Bottom 0.203: TP106.1 | v28.35,67.31 29.36,67.31 30.63,66.04 30.63,61.98 TP106.1 | TP106.1
EZFET_TDI
  Top 0.203: MSP101.61 26.59,66.95 26.19,66.55 26.19,65.66 26.7,65.15 TP104.1 | TP104.1
EZFET_TDO
  Top 0.203: TP103.1 24.16,61.85 26.31,64.01 26.31,65.02 25.81,65.53 25.81,66.87 MSP101.60
EZFET_TEST
  Top 0.203: 25.93,67.69 25.92,67.69 MSP101.59 25.43,67.19 25.43,65.41 25.93,64.9 25.93,64.26 22.5,60.83 TP102.1
EZFET_TMS
  Top 0.203: MSP101.62 26.95,66.55 26.57,66.17 26.57,65.79 27.08,65.28 27.08,62.99 TP105.1
EZFET_UARTRXD  (via drill 0.3)
  Top 0.203: MSP101.38 26.31,75.18 26.31,74.93 26.44,74.8 v26.44,74.3 | J101.5 41.94,59.59 39.19,62.33 39.19,63.48 v39.22,63.5
  Bottom 0.203: v26.44,74.3 30.63,70.1 33.81,70.1 35.2,68.71 35.2,64.64 37.11,62.74 38.46,62.74 v39.22,63.5
EZFET_UARTTXD  (via drill 0.3)
  Top 0.203: MSP101.37 26.25,75.89 v26.95,75.18 | v38.23,63.5 38.23,62.76 39.4,61.59 J101.7
  Bottom 0.203: v26.95,75.18 27.08,74.17 30.76,70.48 33.93,70.48 35.59,68.83 35.59,64.77 37.24,63.12 37.85,63.12 v38.23,63.5
EZFET_V18
  Top 0.203: MSP101.55 24.45,69.05 23.22,67.82 22.12,67.82 19.22,64.91 C102.1
EZFET_VBUS  (via drill 0.3)
  Top 0.203: 9.3,73.28 9.3,73.15 IC102.6 | 9.55,73.28 IC102.6 | IC102.6 | 51.1,77.75 51.1,78.02 C109.+
  Top 0.254: IC103.2 50.32,63.5
  Top 0.305: MSP101.53 23.11,69.11 19.61,69.11 17.3,66.8 13.36,66.8 11.71,65.15 11.33,65.15 | 19.33,71.88 IC101.1 IC101.6 | 51.06,73.75 51.06,74.92 C118.1 51.11,75.99 R120.1
  Top 0.406: 50.32,63.5 C125.1 49.3,63.5
  Top 0.508: 9.3,75.18 9.3,73.28 | 9.55,73.28 v10.69,73.79 | 9.3,75.18 7.14,75.18 5.99,74.04 5.99,70.46 11.33,65.15 11.46,64.97 R124.1 10.48,65.06 9.8,64.39 9.8,59.94 11.33,58.42 29.74,58.42 30.96,59.64 33.1,59.64 J101.11 | v18.31,73.79 18.69,74.17 18.69,74.42 19.08,74.8 19.04,74.8 C108.1 19.37,74.76 19.96,74.17 19.96,72.52 19.33,71.88 | J102.1 9.39,75.28 9.3,75.18 | 51.1,77.75 51.1,76.1 51.06,76.05 R120.1 | 51.06,74.97 C118.1 | 51.06,73.75 C117.1 51.03,73.71 51.59,73.15 51.59,72.52 51.61,72.52 v51.64,72.54 | T101.2 49.32,70.47 | 49.32,70.47 49.3,70.48 | v49.33,70.43 49.33,70.46 49.32,70.47 | v49.05,65.02 49.3,64.77 49.3,63.54 C125.1
  Top 0.635: C109.+ 50.62,77.97 50.39,77.95 v49.48,77.95
  Bottom 0.305: 48.87,77.9 48.74,77.95
  Bottom 0.508: v10.69,73.79 v18.31,73.79 20.47,75.95 20.47,79.88 22.38,81.79 44.86,81.79 48.74,77.95 v49.48,77.95 | v51.64,72.54 50.62,72.54 49.33,71.25 v49.33,70.43 49.33,69.11 48.03,67.82 48.03,66.04 v49.05,65.02
EZFET_VCC  (via drill 0.3)
  Top 0.152: MSP101.11 32.03,69.47 32.07,69.43 | 33.86,68.89 C114.1 | 33.43,70.87 MSP101.15
  Top 0.203: 24.66,75.41 MSP101.40 | R116.1 27.08,81.53 | C114.1 34.06,69.22 | 33.86,68.89 34.13,69.15 | 34.95,76.83 34.98,76.86 | R109.2 32.6,64.4 v32.79,64.47
  Top 0.254: 17.93,71.63 IC101.3 | IC103.4 51.59,62.48 | C103.1 23.1,76.36 23.05,76.41
  Top 0.305: MSP101.40 25.19,74.92 24.28,75.82 C103.1 | 25.52,81.44 R117.1 25.44,81.41 | 46.17,81.82 C124.1 46.04,81.3 45.99,81.19 | 48.14,79.81 C106.+ | 43.59,80.9 45.69,80.9 45.99,81.19 | 38.42,78.92 38.38,79.12 38.38,79.63 39.14,80.39 41.3,80.39 43.46,78.23 46.76,78.23 47.56,79.03 C106.+ | 38.42,78.92 38.43,78.84 | 33.6,70.71 MSP101.15 | 32.07,69.43 32.66,68.83 v32.92,68.83 33.76,68.83 34.13,69.15 35.08,70.1 | v37.11,78.79 37.64,78.79 MSP102.16 MSP102.15 38.42,78.92 | C106.+ 47.73,79.47 47.9,79.68 v47.9,80.9 | 46.06,81.14 45.99,81.19 | 35.08,70.1 35.38,69.93 36.55,69.93 38,71.37 38,72.26 35.46,74.8 35.46,76.33 34.98,76.81 34.98,76.86 v34.98,77.55 | 35.08,70.1 35.14,70.1 C113.1 | 35.08,70.1 34.19,70.1 33.43,70.87 | 23.05,76.41 21.49,77.98 21.49,78.1 C104.+
  Top 0.406: 17.85,71.97 17.93,71.84 17.93,71.63 | 17.42,74.55 17.3,74.55 C105.1 16.88,74.71
  Top 0.508: 16.88,74.71 16.03,75.56 16.03,77.72 16.28,77.98 18.91,77.98 R114.1 21.26,77.94 C104.+ 23.42,78.13 24.03,78.74 24.03,80.77 24.66,81.41 25.44,81.41 27,81.41 R116.1 27.26,81.47 27.97,82.17 42.32,82.17 43.59,80.9 45.62,80.9 46.02,81.23 46.02,81.74 | 17.85,71.97 17.42,72.39 17.42,74.55 17.34,74.76 17.35,74.76 | v47.9,80.9 47.02,81.79 C124.1 | v55.14,61.7 55.14,61.72 54.89,61.47 52.1,61.47 51.59,61.98 51.59,62.48
  Bottom 0.203: v32.92,68.83 32.92,64.59 v32.79,64.47
  Bottom 0.305: v37.11,78.79 36.22,78.79 v34.98,77.55
  Bottom 0.508: v47.9,80.9 49.68,80.9 55.14,75.44 v55.14,61.7
EZFET_VCCEN1  (via drill 0.3)
  Top 0.203: MSP101.26 30.69,75.24 31.14,75.69 32.03,75.69 32.66,76.33 33.55,76.33 34.57,75.31 34.57,74.55 36.32,72.8 v36.32,71.73 | v50.06,62.48 50.32,62.48 50.83,63 IC103.3 | R107.1 43.15,65.97 v43.21,66.29
  Bottom 0.203: v50.06,62.48 49.68,62.48 47.78,64.39 45.11,64.39 v43.21,66.29 43.08,66.42 41.3,66.42 40.54,67.18 40.54,70.87 39.9,71.5 36.55,71.5 v36.32,71.73
EZFET_VCCEN2  (via drill 0.3)
  Top 0.203: MSP101.27 30.76,76.07 31.78,76.07 32.41,76.71 33.81,76.71 34.95,75.56 34.95,74.68 37.11,72.52 v37.11,72.21 | R108.1 v44.35,66.29 | IC103.7 52.47,64 52.73,64.26 v52.73,64.77
  Bottom 0.203: v52.73,64.77 52.48,65.02 50.06,65.02 49.3,64.26 48.54,64.26 48.03,64.77 45.87,64.77 v44.35,66.29 43.71,66.93 41.55,66.93 41.05,67.44 41.05,70.99 39.9,72.14 37.19,72.14 v37.11,72.21
EZFET_VCCOUT
  Top 0.203: 41.81,65.9 40.69,64.77 40.5,64.58 37.27,64.58 36.18,63.48 R121.1 | 41.81,65.9 41.81,65.91 41.94,65.91 42.95,66.93 44.22,66.93 44.73,67.44 44.73,67.47 R127.1 | 41.81,65.9 R112.1 | R128.1 R126.1
  Top 0.254: 51.59,64.52 IC103.8
  Top 0.305: C120.1 45.4,65.54 45.4,67.06 R127.1 44.87,69.29 R128.1 | 46.63,65.57 46.63,65.54
  Top 0.508: 50.55,66.02 50.55,65.56 51.59,64.52
  Top 0.635: 46.63,65.57 47.19,66.02 50.43,66.02 C119.1 50.46,65.99 50.47,65.99 | L101.2 50.44,67.91 50.44,66.27 50.42,66.27 50.42,66.17 50.55,66.17 50.55,66.02 50.47,66.02 50.47,65.99 | 50.47,65.96 50.47,65.99 | 46.63,65.54 C120.1
EZFET_VCCTARGET  (via drill 0.3)
  Top 0.254: IC103.5 52.21,63
  Top 0.305: IC103.1 50.71,64 v50.32,64.39 | 52.21,63 52.6,63 52.73,62.87 v52.73,62.31
  Bottom 0.508: v50.32,64.39 51.59,64.39 52.73,63.25 v52.73,62.31 50.5,60.07 38.51,60.07 J101.9
EZFET_VCORE
  Top 0.203: MSP101.17 34.93,73.16 C101.1
EZFET_VREF
  Top 0.203: C121.1 31.98,66.84 31.98,68.1 MSP101.9
EZFET_VUSB
  Top 0.305: MSP101.54 23.04,68.34 20.36,68.34 20.09,68.07 | C107.1 20.09,68.07 | 20.09,68.07
EZFET_XT2IN
  Top 0.203: MSP101.57 25.16,68.37 24.23,67.41 23.24,67.41 22.06,66.23 22,66.17
  Top 0.406: Q101.1 22.06,66.17 22.06,66.23
EZFET_XT2OUT
  Top 0.203: MSP101.58 24.79,67.27 24.79,64.9 24.2,64.31
  Top 0.406: Q101.3 24.2,64.05 24.2,64.31
GND  (via drill 0.3)
  Top 0.152: v25.17,77.34 25.17,75.56 25.43,75.31 MSP101.39 | MSP102.TP 38.76,78.49 39.14,78.87 MSP102.14 | 26.79,70.14 26.82,70.1 MSP101.TP 27.2,70.74
  Top 0.203: 33.63,71.4 33.53,71.4 | 33.63,71.4 33.63,71.39 MSP101.16 | MSP101.56 24.83,68.75 | MSP101.39 25.93,74.85 25.93,74.7 25.76,74.52 | MSP101.14 32.79,70.81 32.79,71.14 33.1,71.48 33.53,71.48 33.63,71.4 | C101.2 34,74.79 v33.91,74.88
  Top 0.254: 24.83,68.75 24.86,68.75 25.12,69.01 v25.12,70.26 | Q101.2 22.95,64.99 21.62,63.65 | C121.2 32.94,67.41 33.43,66.93
  Top 0.305: 21.62,63.65 18.46,63.63 C102.2
  Bottom 0.203: v20.68,64.41 21.23,64.41 21.72,64.9
  other vias: 10.57,67.82 8.89,68.83 51.08,82.3 41.45,78.87 24.18,66.78 35.33,71.37 19.96,82.55 23.01,75.44 53.49,63.45 43.69,80.04 46.18,66.78 45.75,68.61 47.83,76.33 44.09,73.28 52.7,81.03 17.25,80.14 47.07,82.55 35.59,72.54 48.34,71.12 49.1,74.96 8.43,64.72 16.59,66.07 25.17,78.97 28.85,79.98 17.07,64.85 22.35,62.97 18.95,66.62 27.41,67.46 30.66,73.66 12.22,62.23 22.12,79.65 5.18,72.64 5.23,76.33 16.66,82.42 5.79,79.6 15.72,74.57 13.49,69.34 11.66,74.63 14.88,77.34 16.1,70.48 8.41,71.37 11.46,76.58 27.69,63.91 47.8,72.24 38.4,70.61 41.61,74.24 42.49,67.94 49.76,79.2 21.62,73.53 41.81,71.09 7.9,62.1 1.17,63.37 1.17,72.26 1.17,77.72 21.74,82.55 57.2,60.76 57.48,69.06 57.53,73.66 57.53,77.67 54.69,77.04 56.44,67.18 54.64,60.07 25.43,59.82 30.12,57.66 15.77,59.82 25.91,62.59 6.05,67.18 19.15,73.28 17.3,67.94 26.59,72.14 28.19,70.46 38.15,77.6 39.42,76.71 21.49,71.63 7.21,73.99 12.85,76.58 13.36,72.64 28.91,73.89 53.64,72.67 37.72,69.9 34.04,66.6 52.86,60.5 49.02,67.06 54.05,66.55 50.06,60.91 53.44,65.58 45.67,62.97 51.26,71.12 28.88,75.44 36.12,80.77 42.24,64.74 37.11,61.21 45.39,62.05 42.75,62.18 29.64,63.3 33.96,62.56 31.52,62.48 35.71,60.71
  pour Top: 0.03,57.4 58.45,57.4 58.45,83.82 0.03,83.82
  pour Bottom: 0.03,57.4 58.45,57.4 58.45,83.82 0.03,83.82
  pour MidBottom: 0.03,83.82 58.45,83.82 58.45,57.4 0.03,57.4
N$2
  Top 0.305: R1.2 19.96,40.01 C13.1 24.49,40.1 MSP1.80
N$3
  Top 0.508: J8.2 C1.+
N$4
  Top 0.254: R4.2 36.81,3.3 LED2.A
N$5
  cutout MidBottom: 25.3,38.99 25.3,40.51 24.92,40.89 23.14,40.89 21.87,42.16 21.87,48.01 22.63,48.77 36.09,48.77 37.62,47.24 37.62,43.69 35.59,41.66 28.73,41.66 27.71,40.64 27.71,39.12 27.46,38.86 25.43,38.86
  cutout Top: 25.3,38.99 25.3,40.51 24.92,40.89 23.14,40.89 21.87,42.16 21.87,48.01 22.63,48.77 36.09,48.77 37.62,47.24 37.62,43.69 35.59,41.66 28.73,41.66 27.71,40.64 27.71,39.12 27.46,38.86 25.43,38.86
  cutout MidTop: 25.3,38.99 25.3,40.51 24.92,40.89 23.14,40.89 21.87,42.16 21.87,48.01 22.63,48.77 36.09,48.77 37.62,47.24 37.62,43.69 35.59,41.66 28.73,41.66 27.71,40.64 27.71,39.12 27.46,38.86 25.43,38.86
  cutout Bottom: 25.3,38.99 25.3,40.51 24.92,40.89 23.14,40.89 21.87,42.16 21.87,48.01 22.63,48.77 36.09,48.77 37.62,47.24 37.62,43.69 35.59,41.66 28.73,41.66 27.71,40.64 27.71,39.12 27.46,38.86 25.43,38.86
N$6
  Top 0.254: 15.27,5.29 arc-90 R3.1 15.27,5.29 | J7.2 15.27,5.29
N$7
  Top 0.254: LED1.A 13.88,3.56 R3.2
N$8
  Top 0.254: MSP1.78 25.49,40.58 23.06,43 Q1.2 23.14,43.76 C7.1
N$9
  Top 0.203: 32.66,79.12 32.82,79.27 | 32.82,79.27 32.92,79.38 | R101.1 32.66,79.38 | 32.66,79.38 | 32.82,79.27 LED101.A 32.66,79.36 32.66,79.38
N$10
  Top 0.254: MSP1.74 27.49,41.18 28.47,42.16 31.52,42.16 32.79,43.43 32.79,44.7 | 32.79,44.7 33.05,44.7 | 33.05,44.7 Q2.2 | 33.21,44.74 33.05,44.7 | C9.1 34.15,47.34 32.79,45.97 32.79,44.7
N$11
  Top 0.254: MSP1.75 26.99,41.44 28.22,42.67 30.25,42.67 30.76,43.18 30.76,44.7 | 30.76,44.7 Q2.1 | 30.34,45.12 30.63,44.83 | 30.63,44.83 30.76,44.7 | C8.1 29.4,47.34 30.76,45.97 30.76,44.96 30.63,44.83
N$12
  Top 0.305: T102.2 46.78,71.49 46.76,71.5 45.87,71.5 45.53,71.84 R119.1
N$13
  Top 0.254: T102.1 D101.2 D101.1 46.27,76.98 45.87,76.58 44.98,76.58 R118.1
  Top 0.305: R118.1 44.79,76.59
N$14
  Top 0.254: MSP1.77 25.99,41.1 24.97,42.11 Q1.1 24.92,43.74 C6.1
N$15
  Top 0.635: L101.1 53.23,68.74 53.23,68.83 | 53.23,68.83 53.24,69.85 53.24,70.36 52.48,71.12 T101.3 | D102.3 48.68,69.1 49.17,69.6 52.35,69.6 53.11,68.83 53.23,68.83
N$16
  Top 0.203: T102.3 48.8,72.13 48.29,72.64 48.29,75.82 48.79,76.33 49.68,76.33 49.96,76.05 R120.2 | T101.1 50.38,71.82 50.06,72.14 T102.3 | 48.79,72.14 T102.3
  Top 0.406: 48.79,76.33 D101.3
N$17
  Top 0.508: R6.2 44.86,17.78 J8.3
N$20
  Top 0.203: R102.1 32.14,80.5 32.73,81.09 | 32.73,81.09 32.79,81.15 | LED102.A 32.76,81.06 32.73,81.09
P1.0_LED1
  Top 0.254: MSP1.1 24.49,37.77 25.93,36.32 25.93,28.96 14.76,17.78 14.76,10.67 J7.1
P1.1_LED2  (via drill 0.3)
  Top 0.254: MSP1.2 24.22,37.27 25.43,36.07 25.43,29.21 13.74,17.53 v13.74,13.72 | v44.48,4.57 44.48,3.57 R4.1
  Bottom 0.254: v13.74,13.72 14.25,13.72 18.57,9.4 39.65,9.4 v44.48,4.57
P1.2_A2_J1.2
  Top 0.305: MSP1.3 18.63,36.77 13.49,41.91 7.65,41.91 J1.2
P1.3_A3_J1.6
  Top 0.305: MSP1.16 11.16,30.27 9.68,31.75 7.65,31.75 J1.6
P1.4_A4_J3.27
  Top 0.305: MSP1.17 9.63,29.77 J3.27
P1.5_A5_J3.28
  Top 0.305: MSP1.18 10.25,29.27 J3.28
P1.6_SD_MOSI  (via drill 0.3)
  Top 0.254: SD1.3 26.13,17.72 v26.44,18.03 | v28.47,22.1 v28.47,24.38 | v30,31.24 32.03,33.27 MSP1.51
  Bottom 0.254: v26.44,18.03 27.2,18.03 28.73,19.56 28.73,21.84 v28.47,22.1 | v28.47,24.38 28.47,25.65 29.49,26.67 29.49,30.73 v30,31.24
P1.7_SD_MISO  (via drill 0.3)
  Top 0.254: MSP1.52 28.97,33.77 27.46,32.26 27.46,28.45 v27.71,28.19 | v24.92,23.62 22.38,23.62 21.62,22.86 21.62,16.91 SD1.7
  Bottom 0.254: v27.71,28.19 27.71,26.92 24.92,24.13 v24.92,23.62
P2.0_BCLUART_TXD  (via drill 0.3)
  Top 0.254: J101.6 40.16,54.1 40.16,43.94 v39.65,43.43 | v32.54,29.72 33.99,28.27 MSP1.41
  Bottom 0.254: v39.65,43.43 38.38,43.43 34.06,39.12 33.05,39.12 31.52,37.59 31.52,30.73 v32.54,29.72
P2.1_BCLUART_RXD  (via drill 0.3)
  Top 0.254: J101.8 39.4,44.45 38.89,43.94 v38.89,42.42 | v33.81,29.72 34.76,28.77 MSP1.42
  Bottom 0.254: v38.89,42.42 37.87,41.4 37.11,41.4 34.06,38.35 33.3,38.35 32.28,37.34 32.28,31.24 v33.81,29.72
P2.2_SD_SPICLK  (via drill 0.3)
  Top 0.254: MSP1.43 35.27,29.27 34.06,30.48 28.98,30.48 28.47,29.97 v28.47,28.96 | SD1.5 23.93,18.01 22.12,19.81 22.12,22.5 22.48,22.86 25.43,22.86 v26.95,24.38
  Bottom 0.254: v28.47,28.96 28.47,26.67 26.95,25.15 v26.95,24.38
P2.5_IO_J4.34  (via drill 0.3)
  Top 0.254: MSP1.35 31.49,23.4 32.54,22.35 42.95,22.35 44.73,24.13 44.73,27.69 v46,28.96
  Bottom 0.254: v46,28.96 48.03,28.96 J4.34
P2.6_CAPTURE_J4.35  (via drill 0.3)
  Top 0.254: MSP1.36 31.99,23.67 32.79,22.86 42.7,22.86 44.22,24.38 44.22,28.19 v44.98,28.96
  Bottom 0.254: v44.98,28.96 45.75,29.72 46.76,29.72 49.56,32.51 J4.35
P3.0_A12_J3.23
  Top 0.305: MSP1.4 18.11,36.27 13.74,40.64 J3.23
P3.1_A13_J3.24
  Top 0.305: MSP1.5 17.6,35.77 15.27,38.1 J3.24
P3.2_A14_J3.25
  Top 0.254: 17.33,35.27 16.28,36.32 9.68,36.32 J3.25
  Top 0.305: MSP1.6 17.33,35.27
P3.3_A15_J3.26
  Top 0.305: MSP1.7 17.07,34.77 16.03,35.81 11.71,35.81 J3.26
P3.4_PWM_J4.37
  Top 0.254: MSP1.47 44.5,31.27 47.78,34.54 47.78,36.32 J4.37
P3.5_PWM_J4.38
  Top 0.254: MSP1.48 44.24,31.77 47.27,34.8 47.27,38.35 J4.38
P3.6_PWM_J4.39
  Top 0.254: MSP1.49 43.98,32.27 46.76,35.05 46.76,40.39 J4.39
P3.7_PWM_J4.40
  Top 0.254: MSP1.50 43.72,32.77 46.25,35.31 46.25,42.42 J4.40
P4.0_SD_CS
  Top 0.254: SD1.2 27.23,17.66 R5.1 28.84,18.91 29.49,19.55 MSP1.31
P4.1_IO_J4.31
  Top 0.254: MSP1.32 29.99,22.62 31.78,20.83 43.71,20.83 45.75,22.86 J4.31
P4.2_IO_J4.32  (via drill 0.3)
  Top 0.254: MSP1.33 30.49,22.88 32.03,21.34 43.46,21.34 45.75,23.62 45.75,24.89 v46.25,25.4
  Bottom 0.254: v46.25,25.4 J4.32
P4.3_IO_J4.33  (via drill 0.3)
  Top 0.254: 46,27.94 v46.25,27.94 45.24,26.92 45.24,23.88 43.21,21.84 32.28,21.84 30.99,23.14 MSP1.34
  Bottom 0.254: v46.25,27.94 J4.33
P4.4_IO_J2.18  (via drill 0.3)
  Top 0.254: MSP1.57 43.66,36.27 v44.98,37.59
  Bottom 0.254: v44.98,37.59 46.76,39.37 50.83,39.37 J2.18
P4.7_IO_J3.29  (via drill 0.3)
  Top 0.254: MSP1.12 15.25,32.27 v14.76,32.77 | v14.5,26.67 10.19,26.67 J3.29
  Bottom 0.254: v14.76,32.77 14.76,26.92 v14.5,26.67
P5.0_SPIMOSI_J2.15  (via drill 0.3)
  Top 0.254: MSP1.53 43.95,34.27 v44.22,34.54
  Bottom 0.254: v44.22,34.54 44.48,34.29 50.83,34.29 J2.15
P5.1_SPIMISO_J2.14  (via drill 0.3)
  Top 0.254: MSP1.54 42.67,34.77 v42.95,35.05 | v48.03,32.77 48.03,32.26 48.54,31.75 50.83,31.75 J2.14
  Bottom 0.254: v42.95,35.05 42.95,34.54 43.97,33.53 47.27,33.53 v48.03,32.77
P5.2_SPICLK_J1.7  (via drill 0.3)
  Top 0.254: v27.97,34.04 29.2,35.27 MSP1.55
  Bottom 0.254: J1.7 6.88,30.48 8.15,31.75 11.46,31.75 13.23,33.53 14.25,33.53 14.76,34.04 v27.97,34.04
P5.3_IO_J2.17  (via drill 0.3)
  Top 0.254: MSP1.56 44.69,35.77 v45.24,36.32
  Bottom 0.254: v45.24,36.32 48.29,36.32 48.79,36.83 50.83,36.83 J2.17
P5.5_BUTTON2  (via drill 0.3)
  Top 0.254: MSP1.66 31.49,38.32 v30.76,37.59
  Bottom 0.254: v30.76,37.59 30.76,25.15 35.59,20.32 49.56,20.32 S2.1
P5.6_BUTTON1  (via drill 0.3)
  Top 0.254: MSP1.67 30.99,38.83 30.76,38.61 30.51,38.61 v29.49,37.59
  Bottom 0.254: v29.49,37.59 29.49,32 15.27,17.78 S1.1
P5.7_PWM_J2.19  (via drill 0.3)
  Top 0.254: MSP1.68 30.49,40.62 30.76,40.89 35.33,40.89 36.09,41.66 v45.24,41.66
  Bottom 0.254: v45.24,41.66 45.49,41.91 50.83,41.91 J2.19
P6.0_UTXD_J1.4  (via drill 0.3)
  Top 0.254: J1.4 7.65,36.83 9.68,36.83 10.19,37.34 v14.25,37.34 | MSP1.8 16.94,34.27 16.15,35.05 v14.76,35.05
  Bottom 0.254: v14.76,35.05 14.76,36.83 v14.25,37.34
P6.1_URXD_J1.3  (via drill 0.3)
  Top 0.254: MSP1.9 16.8,33.77 16.28,34.29 14,34.29 v13.74,34.54 | J1.3 7.65,39.37 12.73,39.37 v13.23,38.86
  Bottom 0.254: v13.74,34.54 13.74,36.32 13.23,36.83 v13.23,38.86
P6.2_IO_J1.5  (via drill 0.3)
  Top 0.254: MSP1.10 16.54,33.27 16.03,33.78 11.2,33.78 v10.95,34.04
  Bottom 0.254: v10.95,34.04 10.69,34.29 7.65,34.29 J1.5
P6.3_IO_J1.8  (via drill 0.3)
  Top 0.254: MSP1.11 16.02,32.77 v15.77,33.02 | v15.52,27.43 10.19,27.43 9.42,26.67 7.65,26.67 J1.8
  Bottom 0.254: v15.77,33.02 15.77,27.69 v15.52,27.43
P7.0_I2CSDA_J1.10  (via drill 0.3)
  Top 0.254: MSP1.13 13.98,31.77 v13.74,32
  Bottom 0.254: v13.74,32 13.74,25.65 9.68,21.59 7.65,21.59 J1.10
P7.1_I2CSCL_J1.9  (via drill 0.3)
  Top 0.254: MSP1.14 12.95,31.27 v12.73,31.5 | v11.2,24.13 7.65,24.13 J1.9
  Bottom 0.254: v12.73,31.5 12.73,25.65 v11.2,24.13
P7.2_SD_DETECT
  Top 0.254: SD1.B 17.81,6.67 17.81,10.92 16.54,12.19 R7.2 16.17,13.07 15.52,13.72 15.52,17.53 22.5,24.51 25.81,24.51 26.49,25.19 MSP1.25
P7.3_CAPTURE_J4.36  (via drill 0.3)
  Top 0.254: v42.7,37.08 v37.87,37.08 | MSP1.26 26.99,35.34 28.47,36.83 v33.55,36.83
  Bottom 0.254: J4.36 44.22,35.56 v42.7,37.08 | v37.87,37.08 33.81,37.08 v33.55,36.83
P8.0_IO_J3.30  (via drill 0.3)
  Top 0.254: MSP1.15 11.93,30.77 v11.71,30.99
  Bottom 0.254: v11.71,30.99 11.71,25.65 J3.30
P8.1_IO_J2.11
  Top 0.254: MSP1.44 46.2,29.77 47.52,28.45 47.52,25.4 48.79,24.13 50.83,24.13 J2.11
P8.2_IO_J2.12
  Top 0.254: MSP1.45 46.46,30.27 48.03,28.7 48.03,27.43 48.79,26.67 50.83,26.67 J2.12
P8.3_IO_J2.13
  Top 0.254: MSP1.46 46.73,30.77 48.29,29.21 50.83,29.21 J2.13
TEST/SBWTCK  (via drill 0.3)
  Top 0.254: MSP1.37 32.49,23.93 33.05,23.37 42.19,23.37 v42.44,23.62 | v53.62,24.13 57.18,27.69 57.18,52.83 55.65,54.36 48.54,54.36 J101.2
  Bottom 0.254: v42.44,23.62 47.78,23.62 48.29,24.13 v53.62,24.13
TGT_GND  (via drill 0.3)
  Top 0.254: MSP1.79 24.99,38.54 25.17,38.35 v25.81,38.35 26.31,38.35 26.49,38.52 MSP1.76 | MSP1.73 27.99,38.76 v27.58,38.35 | MSP1.39 33.49,27.63 v33.43,27.69 | MSP1.60 36.4,37.77 v36.98,38.35 36.35,38.99 C4.2 | C7.2 23.14,47.12 | C6.2 24.92,47.12 | MSP1.19 23.33,28.77 v24.03,29.46
  Top 0.61: C9.2 v31.78,47.88 C8.2 | 23.14,47.12 v24.03,48.01 24.92,47.12
  MidBottom 0.203: v31.78,47.88 v31.78,49.4 | v24.03,48.01 v24.03,49.53
  other vias: 13.23,52.58 17.2,2.03 30.02,51.44 8.15,8.64 8.15,6.35 8.15,3.81 7.26,11.3 11.2,10.41 11.96,6.35 20.6,14.73 33.55,1.91 19.33,42.04 18.95,38.61 24.28,19.05 18.95,25.91 37.49,25.65 38.4,52.7 37.64,48.9 19.86,50.93 26.47,55.24 23.27,20.07 22.76,18.03 30.12,14.73 25.3,4.57 51.87,55.5 42.98,51.94 53.64,51.44 40.94,39.24 11.73,48.9 1.83,54.23 3.35,41.53 3.35,29.08 2.08,7.49 12.5,20.45 31.55,18.92 55.93,10.03 55.42,31.62 55.17,41.78 41.2,27.81
  pour Top: 0.03,56.64 0.03,0 58.45,0 58.45,56.64
  pour MidBottom: 0.03,56.64 0.03,0 58.45,0 58.45,56.64
  pour Bottom: 0.03,56.64 0.03,0 58.45,0 58.45,56.64

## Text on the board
tPlace: RST | P5.6 | P5.5 | P1.0 | P1.1
tNames: microSD
tDocu: IC103 | eZ-FET Rev1.3 | Rev1.1 | MSP430FR5994 | MSP-EXP430FR5994 | RXD << | TXD >> | SBWTDIO | SBWTCK | P3.7 | P1.2 | P3.6 | P5.7 | P6.1 | P3.5 | P3.0 | P4.4 | P6.0 | P3.4 | P3.1 | P5.3 | P6.2 | P7.3 | P3.2 | !RST | P1.3 | P2.6 | P3.3 | P5.0 | P5.2 | P2.5 | P1.4 | P5.1 | P6.3 | P4.3 | P1.5 | P8.3 | P7.1 | P4.2 | P4.7 | P8.2 | P7.0 | P4.1 | P8.0 | P8.1 | Supercap C1 | Use | Charge
tSilk: J | C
